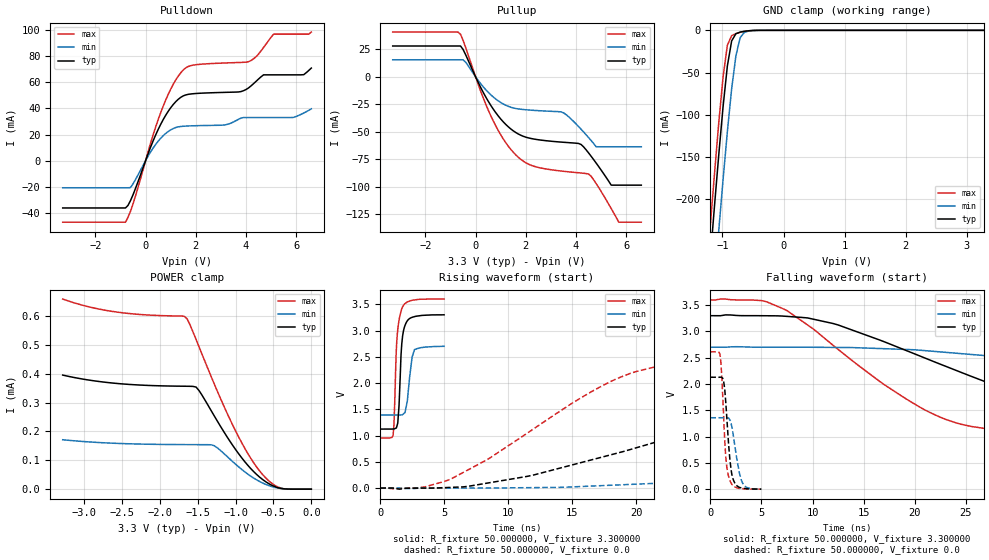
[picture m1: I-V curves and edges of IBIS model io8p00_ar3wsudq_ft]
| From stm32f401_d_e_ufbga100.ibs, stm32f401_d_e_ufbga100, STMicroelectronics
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|   Model io8p00_ar3wsudq_ft
[Model]  io8p00_ar3wsudq_ft
Model_type I/O
Polarity   Non-Inverting
Enable   Active-Low
Vinl =   0.990000V
Vinh =   2.310000V
Vmeas =  1.650000V
Cref =   50.000000pF
Rref =   100.000000M
Vref =   0.0V
C_comp   3.843200pF   3.761700pF   3.937000pF
[Temperature Range]   25.000000   0.125000k   -40.000000
[Pullup Reference]   3.300000V   2.700000V   3.600000V
[Pulldown Reference]   0.0V   0.0V   0.0V
[POWER Clamp Reference]   3.300000V   2.700000V   3.600000V
[GND Clamp Reference]   0.0V   0.0V   0.0V
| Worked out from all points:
|   slope of the pulldown table from 0 to 0.495 V, typ, clamps not added: 20.9 ohm
|   slope of the pullup table from 0 to 0.495 V, typ, clamps not added: 22.6 ohm
|   GND clamp passes 1 mA (typ) near -0.62 V on its own axis
|   rising waveform, R_fixture 50.000000, V_fixture 3.300000: 20-80 % time 268ps typ, 350ps min, 282ps max; typ from 1.12 V to 3.3 V
|   rising waveform, R_fixture 50.000000, V_fixture 0.0: 20-80 % time 19.7ns typ, 50.7ns min, 10.4ns max; typ from 0 V to 2.13 V
|   falling waveform, R_fixture 50.000000, V_fixture 3.300000: 20-80 % time 18.5ns typ, 39.7ns min, 11.3ns max; typ from 3.3 V to 1.12 V
|   falling waveform, R_fixture 50.000000, V_fixture 0.0: 20-80 % time 505ps typ, 696ps min, 424ps max; typ from 2.13 V to 0 V
[Pulldown]
|Voltage   I(typ)   I(min)   I(max)
-3.3V     -36.18mA   -20.77mA   -47.07mA
-800mV    -36.18mA   -20.77mA   -47.07mA
-600mV    -30.5mA    -20.52mA   -38.69mA
700mV     31.4mA     19.11mA    41.71mA
1.2V      45.15mA    25.37mA    61.75mA
1.6V      50.35mA    26.5mA     71.06mA
3.1V      52.28mA    27.26mA    74.76mA
4.1V      55.71mA    33.01mA    75.8mA
4.7V      65.73mA    33.01mA    86.69mA
5.1V      65.73mA    33.01mA    96.9mA
6.3V      65.85mA    36.5mA     96.9mA
6.6V      70.91mA    39.71mA    98.45mA
[Pullup]
|Voltage   I(typ)   I(min)   I(max)
-3.3V     28.03mA    15.43mA    40.67mA
-700mV    28.03mA    15.43mA    40.67mA
-400mV    20.31mA    13.47mA    26.93mA
600mV     -25.77mA   -16.23mA   -35.14mA
1.6V      -50.64mA   -28.81mA   -70.96mA
3.5V      -59.53mA   -32.72mA   -85.92mA
4.2V      -61.52mA   -47.62mA   -87.46mA
4.5V      -69.21mA   -55.27mA   -88.43mA
4.8V      -78.37mA   -63.6mA    -97.01mA
5.4V      -98.5mA    -63.6mA    -119.7mA
5.7V      -98.5mA    -63.6mA    -132.2mA
6.6V      -98.5mA    -63.6mA    -132.2mA
[GND_clamp]
|Voltage   I(typ)   I(min)   I(max)
-3.3V     -2.328A    -2.406A    -2.303A
-1.2V     -270.2mA   -361.4mA   -232.1mA
-1.13V    -207.3mA   -298.1mA   -169mA
-1.06V    -146.7mA   -236.2mA   -108.8mA
-990mV    -90.18mA   -176.4mA   -54.96mA
-920mV    -42.21mA   -120mA     -17.68mA
-850mV    -12.57mA   -69.47mA   -6.265mA
-780mV    -3.971mA   -30.01mA   -3.886mA
-710mV    -2.1mA     -8.615mA   -2.382mA
-640mV    -1.148mA   -2.283mA   -1.22mA
-570mV    -524uA     -821.5uA   -476.8uA
3.28V     0A         0A         0A
[POWER_clamp]
|Voltage   I(typ)   I(min)   I(max)
-3.28V    395.3uA    171.3uA    658.7uA
-2.6V     367.1uA    159uA      614.9uA
-1.68V    356.7uA    154.4uA    599.4uA
-1.64V    356.5uA    154.4uA    590.8uA
-1.52V    353.6uA    154.3uA    518.3uA
-1.48V    341.1uA    154.2uA    492.3uA
-1.28V    253.6uA    150.4uA    364.2uA
-960mV    123.1uA    77.56uA    181.6uA
-720mV    50.52uA    32.03uA    76.18uA
-560mV    18.94uA    12.27uA    28.65uA
-440mV    5.104uA    3.69uA     7.327uA
0V        0A         0A         0A
[Ramp]
| variable   typ   min   max
dV/dt_r  1.27740/19.70093n   0.81594/50.77898n   1.56726/10.32856n
dV/dt_f  1.30662/18.47275n   0.78480/39.80018n   1.58789/11.32219n
R_load = 50.000000
[Rising Waveform]
R_fixture= 50.000000
V_fixture= 3.300000
V_fixture_min= 2.700000
V_fixture_max= 3.600000
|time   V(typ)   V(min)   V(max)
0s        1.124V     1.392V     953.5mV
1.001ns   1.126V     1.392V     1.007V
1.071ns   1.127V     1.392V     1.224V
1.331ns   1.207V     1.392V     2.933V
1.461ns   1.553V     1.391V     3.186V
1.632ns   2.573V     1.393V     3.375V
1.732ns   2.868V     1.397V     3.445V
2.112ns   3.185V     1.656V     3.545V
2.673ns   3.265V     2.635V     3.584V
4.985ns   3.3V       2.7V       3.6V
[Rising Waveform]
R_fixture= 50.000000
V_fixture= 0.0
V_fixture_min= 0.0
V_fixture_max= 0.0
|time   V(typ)   V(min)   V(max)
0s        7.576nV    344.7nV    5.15nV
5.506ns   13.32mV    -139.8uV   170.6mV
16.52ns   537.7mV    38.12mV    1.837V
20.02ns   767.9mV    74.66mV    2.221V
34.53ns   1.706V     287.7mV    2.56V
41.04ns   1.911V     402.5mV    2.582V
57.56ns   2.068V     709.2mV    2.607V
88.09ns   2.119V     1.131V     2.612V
114.6ns   2.127V     1.29V      2.612V
249.2ns   2.129V     1.359V     2.612V
[Falling Waveform]
R_fixture= 50.000000
V_fixture= 3.300000
V_fixture_min= 2.700000
V_fixture_max= 3.600000
|time   V(typ)   V(min)   V(max)
0s        3.3V       2.7V       3.6V
5.506ns   3.299V     2.7V       3.564V
12.01ns   3.151V     2.696V     2.736V
22.02ns   2.414V     2.619V     1.41V
25.53ns   2.146V     2.562V     1.193V
31.03ns   1.755V     2.445V     1.08V
38.54ns   1.415V     2.267V     1.021V
46.55ns   1.276V     2.09V      998mV
84.58ns   1.149V     1.538V     957.1mV
249.2ns   1.124V     1.392V     953.5mV
[Falling Waveform]
R_fixture= 50.000000
V_fixture= 0.0
V_fixture_min= 0.0
V_fixture_max= 0.0
|time   V(typ)   V(min)   V(max)
0s        2.129V     1.359V     2.612V
981ps     2.13V      1.359V     2.52V
1.151ns   2.121V     1.358V     2.041V
1.311ns   2.041V     1.358V     1.357V
1.522ns   1.636V     1.36V      601.2mV
1.902ns   599.4mV    1.321V     175.8mV
2.292ns   159.9mV    969.7mV    55.32mV
2.853ns   34.57mV    304.7mV    13.74mV
3.173ns   16.36mV    110.8mV    9.034mV
4.985ns   7.576nV    344.7nV    5.15nV
